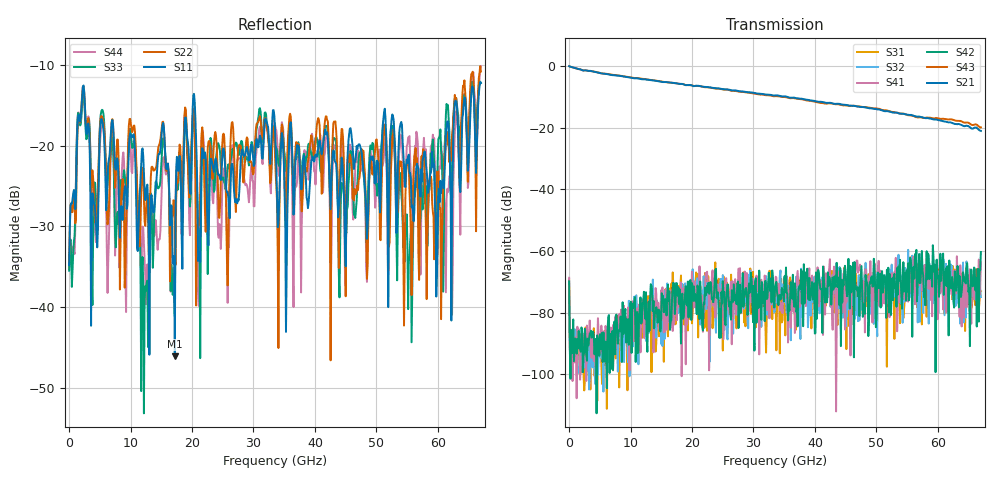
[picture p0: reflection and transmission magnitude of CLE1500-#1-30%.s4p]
!Keysight Technologies,N5247B,US50470101,A.16.20.02
!Date: Thursday, March 13, 2025 10:16:18
!Correction: S11(C  4-Port  )
!S12(C  4-Port  )
!S13(C  4-Port  )
!S14(C  4-Port  )
!S21(C  4-Port  )
!S22(C  4-Port  )
!S23(C  4-Port  )
!S24(C  4-Port  )
!S31(C  4-Port  )
!S32(C  4-Port  )
!S33(C  4-Port  )
!S34(C  4-Port  )
!S41(C  4-Port  )
!S42(C  4-Port  )
!S43(C  4-Port  )
!S44(C  4-Port  )
!S4P File: Measurements: <S11,S12,S13,S14>,
!<S21,S22,S23,S24>,
!<S31,S32,S33,S34>,
!<S41,S42,S43,S44>:
# Hz S  dB  R 50
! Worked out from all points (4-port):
!   601 points, 10 MHz to 67 GHz, reference 50 ohm
!   strongest paths, dB at 10 MHz, 16.76 GHz, 33.51 GHz, 50.25 GHz, 67 GHz:
!     S21: 0.0, -5.4, -9.5, -14.0, -21.0
!     S43: 0.0, -5.4, -9.7, -13.8, -19.8
!     S42: -69.8, -75.5, -72.2, -67.0, -60.3
!     S41: -68.6, -83.3, -76.3, -69.7, -63.6
!     S32: -75.6, -79.9, -78.6, -64.7, -74.9
!     S31: -69.2, -73.2, -79.0, -76.1, -73.0
!   lowest |S11| = -46.1 dB at 17.2 GHz (marker M1), VSWR 1.01, Z = 49.9 + j0.489 ohm
!   |S11| at or under -10 dB: start of sweep to end of sweep
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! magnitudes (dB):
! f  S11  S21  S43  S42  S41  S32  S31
! 10 MHz  -34.8  0.0  0.0  -69.8  -68.6  -75.6  -69.2
! 2.243 GHz  -12.7  -1.4  -1.3  -99.3  -91.0  -89.7  -92.5
! 17.2 GHz  -46.1  -5.4  -5.5  -80.4  -76.2  -71.8  -72.1
! 30.94 GHz  -19.2  -9.0  -9.2  -66.3  -93.5  -80.0  -74.5
! 52.6 GHz  -16.1  -15.0  -14.8  -68.8  -73.5  -74.0  -72.0
! 55.5 GHz  -23.4  -15.8  -16.0  -62.1  -66.9  -74.8  -62.0
! 67 GHz  -12.2  -21.0  -19.8  -60.3  -63.6  -74.9  -73.0
